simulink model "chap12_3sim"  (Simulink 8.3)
settings: Solver=ode45  StartTime=0.0  StopTime=20

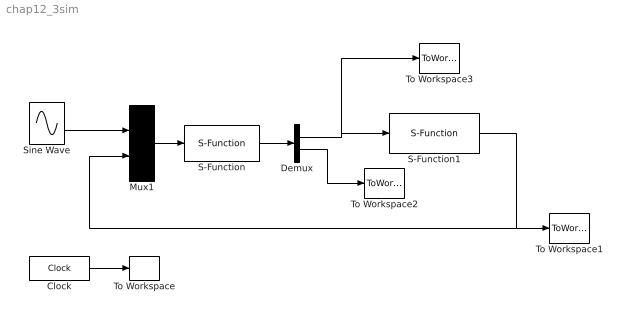
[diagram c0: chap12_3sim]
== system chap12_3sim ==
  Clock : Clock
  Demux : Demux  Outputs=2
  Mux1 : Mux  Inputs=2
  S-Function : S-Function  FunctionName=chap12_3ctrl  EnableBusSupport=off
  S-Function1 : S-Function  FunctionName=chap12_3plant  EnableBusSupport=off
  Sine Wave : Sin  SampleTime=0
  To Workspace : ToWorkspace  VariableName=t  SampleTime=-1
  To Workspace1 : ToWorkspace  VariableName=p  SampleTime=-1
  To Workspace2 : ToWorkspace  VariableName=fxp  SampleTime=-1
  To Workspace3 : ToWorkspace  VariableName=ut  SampleTime=-1
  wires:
  Clock/1 -> To Workspace/1
  Sine Wave/1 -> Mux1/1
  Mux1/1 -> S-Function/1
  S-Function1/1 -> To Workspace1/1, Mux1/2
  S-Function/1 -> Demux/1
  Demux/1 -> To Workspace3/1, S-Function1/1
  Demux/2 -> To Workspace2/1
